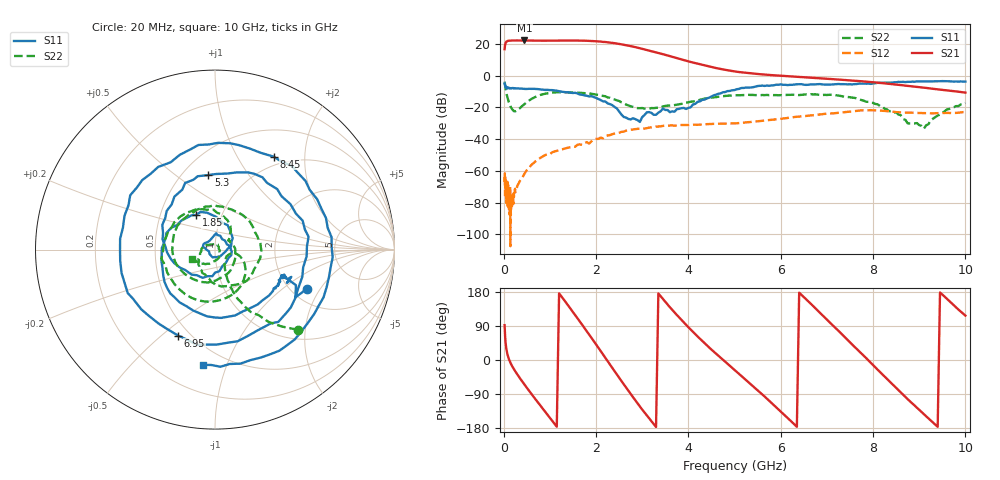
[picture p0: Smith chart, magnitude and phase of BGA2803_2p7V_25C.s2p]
#  HZ  S  RI  R  50.0000
! Rohde & Schwarz ZVA/B
! Temperature 25C
! Device number 102
! Measured Vcc 2.700000
! Measured Icc 0.004700
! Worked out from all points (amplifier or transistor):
!   242 points, 20 MHz to 10 GHz, reference 50 ohm
!   highest |S21| = 22.1 dB at 450 MHz (marker M1)
!   |S21| within 3 dB of that: 28.81 MHz to 2.659 GHz (2.63 GHz wide, 196 % of centre)
!   unconditionally stable (mu >= 1): start of sweep to end of sweep
!   at 220 MHz: K = 166.23, MAG = 22.9 dB, |S12| = -74.1 dB
!   at 4 GHz: K = 6.27, MAG = 9.1 dB, |S12| = -31.1 dB
!   at 10 GHz: K = 13.80, MAG = -8.3 dB, |S12| = -22.9 dB
!   S11 on the Smith chart (normalised r, x): 20 MHz: 2.42, -1.53; 1.85 GHz: 0.75, +0.31; 5.3 GHz: 0.66, +0.67; 6.95 GHz: 0.43, -0.57; 8.45 GHz: 0.87, +1.44; 10 GHz: 0.38, -0.83
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2e7  0.5124 -0.2183  -0.2251 6.766  0.000264 0.000358  0.4614 -0.4473
5e7  0.4037 -0.1646  9.192 6.503  0.000207 -0.000189  0.145 -0.293
1e8  0.383 -0.1562  12.38 1.441  6.52e-05 8.15e-05  0.0653 -0.1512
2.45e8  0.3229 -0.2295  11.13 -6.159  -0.000238 0.00013  0.0641 -0.0388
4.5e8  0.1899 -0.3295  5.405 -11.53  -0.000616 0.000539  0.1228 -0.0252
7.5e8  -0.0457 -0.3714  -4.961 -11.52  4.43e-06 0.00233  0.1605 -0.1668
1.15e9  -0.2809 -0.1809  -12.54 -0.8588  0.0035 0.00242  -0.0958 -0.2828
1.4e9  -0.2966 0.00847  -10.16 7.576  0.00535 0.000741  -0.2468 -0.1602
1.7e9  -0.1894 0.1599  -0.6565 12.53  0.00629 -0.00206  -0.2766 0.0597
1.85e9  -0.1062 0.1932  4.732 11.35  0.00634 -0.00339  -0.2257 0.1539
2.2e9  0.0704 0.1364  11.31 1.257  0.00653 -0.0106  -0.00841 0.2225
2.6e9  0.0431 -0.0249  4.107 -8.372  -0.00553 -0.0161  0.0885 0.1023
2.95e9  -0.033 -0.0107  -3.926 -6.085  -0.0192 -0.00948  0.0781 0.052
3.35e9  -0.0151 0.0662  -5.129 0.4014  -0.0235 0.00814  0.0939 0.0284
4.2e9  -0.0149 -0.1482  1.105 2.082  0.0119 0.0255  0.0233 -0.1616
5.05e9  -0.2262 0.2951  1.126 -0.6902  0.0297 -0.0108  -0.2375 0.0171
5.3e9  -0.0373 0.4154  0.6319 -1.014  0.025 -0.0232  -0.21 0.1313
6.7e9  0.072 -0.5187  -0.6726 0.5141  -0.0562 0.00356  0.2539 -0.0272
6.95e9  -0.2062 -0.4786  -0.3039 0.7412  -0.0531 0.0321  0.21 -0.1293
8.35e9  0.1962 0.5622  0.3121 -0.4543  0.0728 -0.0171  -0.0752 -0.0069
8.45e9  0.3267 0.5179  0.2031 -0.4929  0.0658 -0.029  -0.0669 0.0132
1e10  -0.0681 -0.6423  -0.1324 0.2586  -0.0686 -0.0211  -0.1259 -0.0545
